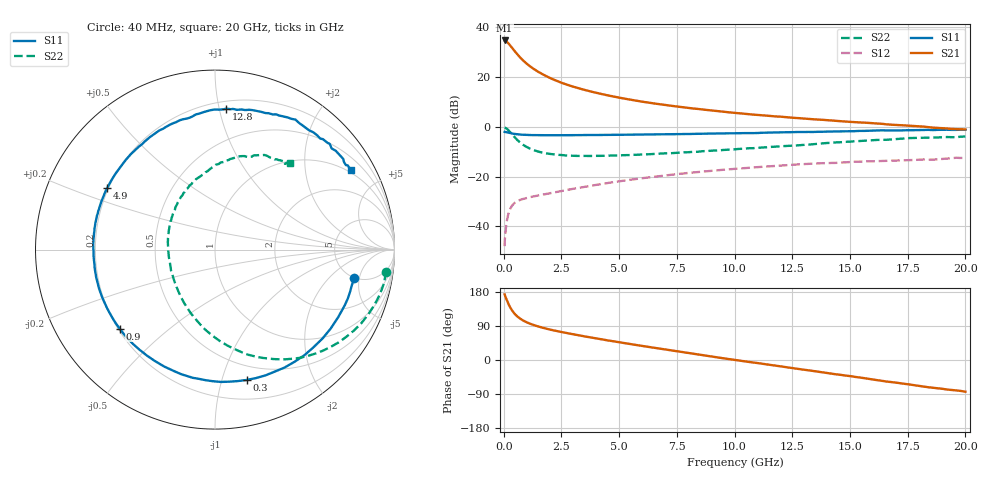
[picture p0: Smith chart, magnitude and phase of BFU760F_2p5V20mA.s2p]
! Filename:  P:\Prog\Test\Noise\ATS_data\Testdata_Net\Split files Spar\BFU760F_2W_C1_Bias5_2.5V_5mA_30mA_D.s2p
! Date/Time: Mon 06/Feb/2012 15:08:18
! BFU760_2W_C1_Bias5_2.5V_5mA_30mA_R.s2p
! MDIF S-parameter v. bias file
! BFU760_2W_C1_2.5V_5mA_30mA
! Date/time Fri Mar 18 11:16:19 2011
! VAR V_out= 2.5000
! VAR I_out= 20.0150
! VAR V_in= 0.7835
! VAR I_in= 0.0612
! Device data file deembeded for feedlines and parallel
! Original file: \Split files Spar\BFU760_2W_C1_Bias5_2.5V_5mA_30mA_R.s2p
! Feed-files: PR003V01_101208_Feed1.s2p, PR003V01_101208_Feed2.s2p
! Parallel-file: PR003V01_101208_Par.s2p
# MHz S MA R 50
!  Freq-MHz  S11-mag  S11-arg  S21-mag  S21-arg  S12-mag  S12-arg  S22-mag  S22-arg
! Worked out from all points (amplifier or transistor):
!   167 points, 40 MHz to 20 GHz, reference 50 ohm
!   highest |S21| = 34.7 dB at 40 MHz (marker M1)
!   |S21| within 3 dB of that: start of sweep to 367.7 MHz
!   unconditionally stable (mu >= 1): 4.28 GHz to 13.62 GHz
!   at 550 MHz: K = 0.25, MSG = 29.9 dB, |S12| = -30.1 dB
!   at 4.2 GHz: K = 1.00, MSG = 18.1 dB, |S12| = -23.0 dB
!   at 20 GHz: K = 0.88, MSG = 5.7 dB, |S12| = -12.5 dB
!   S11 on the Smith chart (normalised r, x): 40 MHz: 4.91, -4.21; 300 MHz: 0.37, -1.20; 900 MHz: 0.21, -0.35; 4.9 GHz: 0.19, +0.26; 12.8 GHz: 0.25, +1.05; 20 GHz: 0.90, +3.48
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40  0.7918 -11.6  54.41 173.2  0.004 73.6  0.9633 -7.4
50  0.7877 -14.7  54.26 171.0  0.005428 75.9  0.9601 -9.5
90  0.7837 -26.1  53.13 164.8  0.00873 73.2  0.9457 -17.3
160  0.7729 -44.7  49.73 154.2  0.01465 66.6  0.8962 -30.2
240  0.7569 -64.0  45.61 143.7  0.02016 59.3  0.8232 -43.2
300  0.7474 -76.3  42.01 137.0  0.02344 54.5  0.7667 -51.9
380  0.7333 -91.0  37.92 129.3  0.0267 49.3  0.6921 -61.8
420  0.7256 -97.1  35.85 126.0  0.02806 47.2  0.6597 -66.2
550  0.7103 -113.5  30.2 117.1  0.03122 42.0  0.5659 -78.7
700  0.6985 -127.1  25.14 109.7  0.03382 38.4  0.4893 -90.1
900  0.6898 -140.3  20.36 102.3  0.0362 35.9  0.418 -102.4
1300  0.6824 -157.0  14.59 92.3  0.04003 34.5  0.3401 -120.8
1850  0.6783 -171.0  10.39 82.6  0.04499 35.1  0.2927 -138.9
2500  0.6791 177.9  7.701 73.9  0.05126 36.5  0.2715 -154.5
3400  0.6827 166.3  5.692 63.5  0.06117 36.9  0.261 -169.9
4900  0.6919 150.3  3.942 47.8  0.07915 34.7  0.2666 169.9
6800  0.7064 133.2  2.827 29.6  0.103 28.1  0.2893 149.8
10200  0.7467 105.4  1.873 -1.4  0.1456 10.7  0.3603 119.2
12800  0.7879 85.4  1.493 -23.8  0.1764 -4.8  0.4265 98.3
13400  0.7883 81.0  1.42 -28.9  0.1824 -9.3  0.4473 94.0
16800  0.8465 55.0  1.103 -58.2  0.2085 -30.8  0.5568 68.4
20000  0.8781 30.3  0.8855 -83.6  0.2372 -52.6  0.639 49.1
